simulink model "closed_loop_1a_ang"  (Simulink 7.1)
settings: Solver=FixedStepDiscrete  StartTime=0.0  StopTime=Tend  FixedStep=Ts  MaxStep=Ts  MinStep=Ts/10  RelTol=1e-4
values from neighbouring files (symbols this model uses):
  Kt = 0.06    [lame_dat.m]
  Ts = 100e-6    (= 0.0001)    [lame_main.m]
undefined symbols (not defined in the file or in its folder): A
libraries: powerlib_extras x1, cstblocks x1

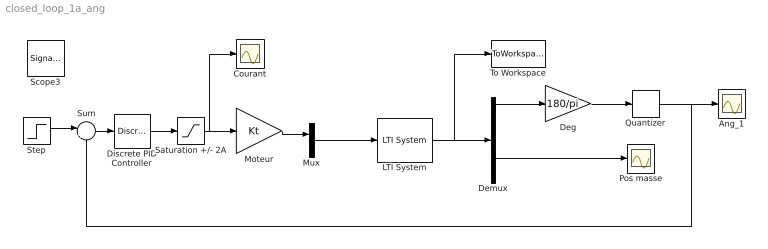
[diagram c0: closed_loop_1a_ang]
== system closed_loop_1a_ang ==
  Ang_1 : Scope
  Courant : Scope
  Deg : Gain  Gain=180/pi  ParameterDataType=fixdt(1, 16)  ParameterScaling=2^0  OutDataType=fixdt(1, 16)  OutScaling=2^0
  Demux : Demux  Outputs=5
  Discrete PID Controller : powerlib_extras/Discrete  Control Blocks/Discrete PID Controller  DialogController=POWERSYS.PowerSysDialog  SystemSampleTime=-1  Kp=10  Ki=50  Kd=0.003  TcD=Ts  Par_Limits="[1    -1]"  Init=0  Ts=Ts
  LTI System : cstblocks/LTI System  SystemSampleTime=-1  sys=sysd  IC=[]
  Moteur : Gain  Gain=Kt  ParameterDataType=sfix(16)  ParameterScaling=2^0  OutDataType=sfix(16)  OutScaling=2^0
  Mux : Mux  Inputs=2
  Pos masse : Scope
  Quantizer : Quantizer  QuantizationInterval=0.1
  Saturation +/- 2A : Saturate  UpperLimit=2  LowerLimit=-2  OutDataType=sfix(16)  OutScaling=2^0
  Step : Step  Time=0  After=A  SampleTime=0
  Sum : Sum  Inputs=|+-  OutDataType=sfix(16)  OutScaling=2^0
  To Workspace : ToWorkspace  VariableName=y_sim_out  SampleTime=-1  SaveFormat=Structure With Time
  Scope3 : SignalViewerScope  IOType=viewer  RefreshTime=0.035000
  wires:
  Deg/1 -> Quantizer/1
  LTI System/1 -> Demux/1, To Workspace/1
  Demux/1 -> Deg/1
  Moteur/1 -> Mux/1
  Mux/1 -> LTI System/1
  Step/1 -> Sum/1
  Sum/1 -> Discrete PID Controller/1
  Discrete PID Controller/1 -> Saturation +/- 2A/1
  Saturation +/- 2A/1 -> Moteur/1, Courant/1
  Quantizer/1 -> Ang_1/1, Sum/2
  Demux/4 -> Pos masse/1
